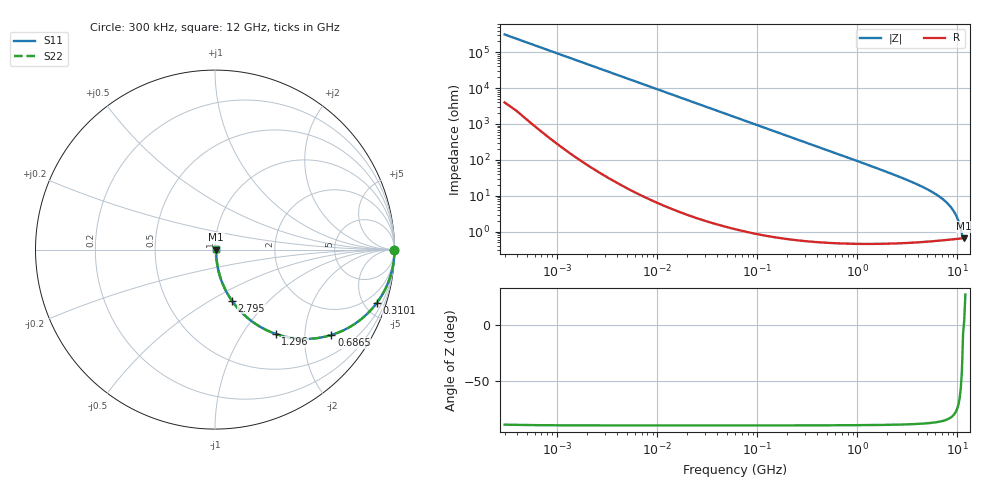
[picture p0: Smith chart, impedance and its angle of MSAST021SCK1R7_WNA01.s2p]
! MSAST021SCK1R7_WNA01  S-PARAMETER MODEL  ( General Type )
! Model Generated by TAIYO YUDEN Corporation (http://www.ty-top.com)
! Version 2.0
! TAIYO YUDEN Control No. 181101
! Copyright(c) 2015 TAIYO YUDEN CO.,LTD. All Rights Reserved.
! Product Description (link to TY-COMPAS)
! https://ds.yuden.co.jp/TYCOMPAS/or/detail?pn=MSAST021SCK1R7BWNA01&u=M
! Products Name : Multilayer Ceramic Capacitors
! Characteristics :
!  Capacitance : 1.7 pF , Rated Voltage : 25V , TCC : CK / C0K
!  Case Size : 0.25 x 0.125 / 0.0098 x 0.0049 [mm/inch] , Thickness : 0.125 / 0.0049 [mm/inch]
!  (Conditions: Temperature = 25 degC , DC Bias Current/Voltage = 0A / 0V)
! External Node Assignments :
!  1  o---| |---o  2
! GND o---------o GND
! Frequency Range : 0.3MHz  -  12000MHz  [ 401 STEP ]
# MHz S RI R 50
! Freq[MHz].  S11 Real  S11 Imag  S21 Real  S21 Imag  S12 Real  S12 Imag  S22 Real  S22 Imag
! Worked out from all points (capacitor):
!   401 points, 300 kHz to 12 GHz, reference 50 ohm
!   read as one part in series: C = 1.7 pF near 316.3 kHz
!   lowest |Z| = 660 mohm at 11.69 GHz (marker M1)
!   series resonance near 11.59 GHz, so ESL is about 110 pH
!   S11 on the Smith chart (normalised r, x): 300 kHz: open; 310.1 MHz: 1.01, -6.03; 686.5 MHz: 1.01, -2.72; 1.296 GHz: 1.01, -1.43; 2.795 GHz: 1.01, -0.63; 12 GHz: 1.01, +0.01
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0.3  1 -0.00032  4.19e-06 0.00032  4.19e-06 0.00032  1 -0.00032
1.769972  1 -0.00189  6.81e-06 0.00189  6.81e-06 0.00189  1 -0.00189
10.44266  0.9999 -0.0112  0.000132 0.0112  0.000132 0.0112  0.9999 -0.0112
60  0.9959 -0.0638  0.00414 0.0638  0.00414 0.0638  0.9959 -0.0638
143.8206  0.9768 -0.1501  0.0232 0.1501  0.0232 0.1501  0.9768 -0.1501
310.0777  0.9006 -0.2983  0.0994 0.2983  0.0994 0.2983  0.9006 -0.2983
353.9943  0.8742 -0.3306  0.1258 0.3306  0.1258 0.3306  0.8742 -0.3306
486.4723  0.7862 -0.4087  0.2138 0.4087  0.2138 0.4087  0.7862 -0.4087
686.4755  0.6482 -0.4758  0.3518 0.4758  0.3518 0.4758  0.6482 -0.4758
943.3804  0.4928 -0.4976  0.5072 0.4976  0.5072 0.4976  0.4928 -0.4976
1296.429  0.338 -0.4698  0.662 0.4698  0.662 0.4698  0.338 -0.4698
2088.533  0.1608 -0.362  0.8392 0.362  0.8392 0.362  0.1608 -0.362
2795.104  0.0938 -0.2841  0.9062 0.2841  0.9062 0.2841  0.0938 -0.2841
5140.631  0.0257 -0.141  0.9743 0.141  0.9743 0.141  0.0257 -0.141
6354.153  0.0157 -0.0999  0.9843 0.0999  0.9843 0.0999  0.0157 -0.0999
7648.807  0.0103 -0.0669  0.9897 0.0669  0.9897 0.0669  0.0103 -0.0669
8503.825  0.00839 -0.0488  0.9916 0.0488  0.9916 0.0488  0.00839 -0.0488
9454.42  0.00715 -0.0313  0.9929 0.0313  0.9929 0.0313  0.00715 -0.0313
10236.47  0.00664 -0.0183  0.9934 0.0183  0.9934 0.0183  0.00664 -0.0183
11083.22  0.00648 -0.00557  0.9935 0.00557  0.9935 0.00557  0.00648 -0.00557
11686.27  0.00654 0.000432  0.9935 -0.000432  0.9935 -0.000432  0.00654 0.000432
12000  0.00661 0.0033  0.9934 -0.0033  0.9934 -0.0033  0.00661 0.0033
